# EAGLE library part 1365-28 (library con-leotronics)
DUAL ROW STRAIGHT HEADER 1364 SERIES. 1.27mm x 1.27mm. Without Fixing Post. SMT Source: http://www.leotronics.co.uk/Conexcon/Data%20Sheets/sec.%20A/1364ing.pdf
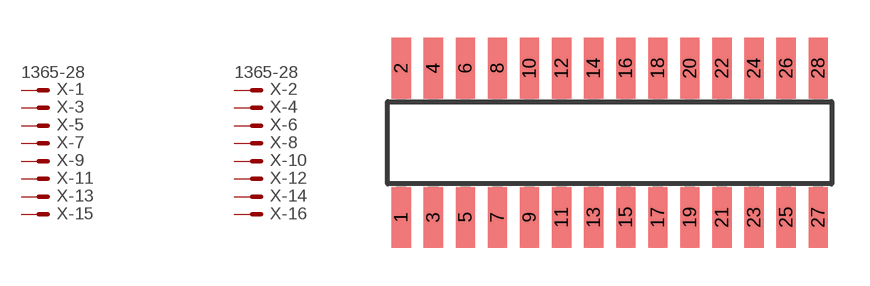
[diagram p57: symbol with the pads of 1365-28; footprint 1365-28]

Designator prefix X; gates -1=MVAL -2=MVAL -3=M -4=M -5=M -6=M -7=M -8=M -9=M -10=M -11=M -12=M -13=M -14=M -15=M -16=M -17=M -18=M -19=M -20=M -21=M -22=M -23=M -24=M -25=M -26=M -27=M -28=M

## 1365-28 (OC_FARNELL: unknown; OC_NEWARK: unknown)  [1365-28]
1  -1:S  pas
2  -2:S  pas
3  -3:S  pas
4  -4:S  pas
5  -5:S  pas
6  -6:S  pas
7  -7:S  pas
8  -8:S  pas
9  -9:S  pas
10  -10:S  pas
11  -11:S  pas
12  -12:S  pas
13  -13:S  pas
14  -14:S  pas
15  -15:S  pas
16  -16:S  pas
17  -17:S  pas
18  -18:S  pas
19  -19:S  pas
20  -20:S  pas
21  -21:S  pas
22  -22:S  pas
23  -23:S  pas
24  -24:S  pas
25  -25:S  pas
26  -26:S  pas
27  -27:S  pas
28  -28:S  pas

## Footprint 1365-28 (pad centres in mm)
DUAL ROW STRAIGHT HEADER 1364 SERIES. 1.27mm x 1.27mm. Without Fixing Post. SMT Source: http://www.leotronics.co.uk/Conexcon/Data%20Sheets/sec.%20A/1364ing.pdf
smd 0.76 x 2.4: 1 -8.255,-2.95; 2 -8.255,2.95; 3 -6.985,-2.95; 4 -6.985,2.95; 5 -5.715,-2.95; 6 -5.715,2.95; 7 -4.445,-2.95; 8 -4.445,2.95; 9 -3.175,-2.95; 10 -3.175,2.95; 11 -1.905,-2.95; 12 -1.905,2.95; 13 -0.635,-2.95; 14 -0.635,2.95; 15 0.635,-2.95; 16 0.635,2.95; 17 1.905,-2.95; 18 1.905,2.95; 19 3.175,-2.95; 20 3.175,2.95; 21 4.445,-2.95; 22 4.445,2.95; 23 5.715,-2.95; 24 5.715,2.95; 25 6.985,-2.95; 26 6.985,2.95; 27 8.255,-2.95; 28 8.255,2.95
